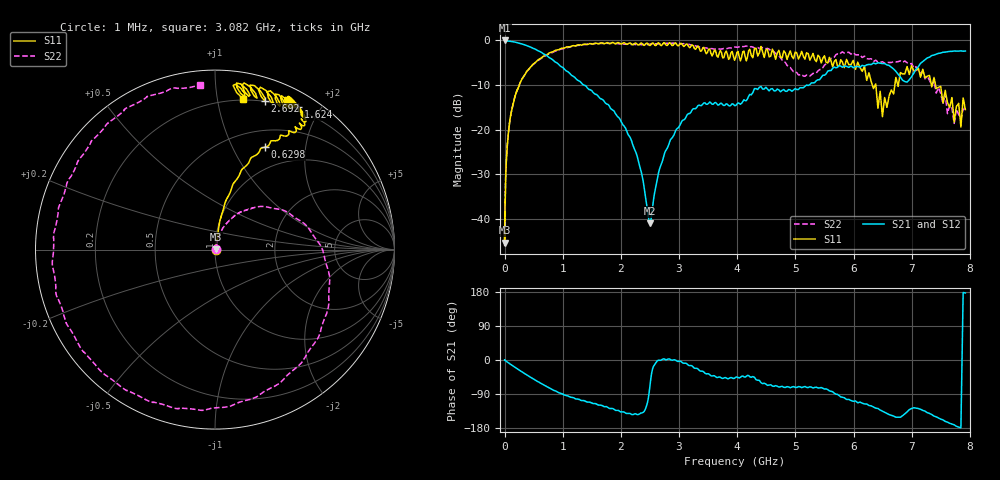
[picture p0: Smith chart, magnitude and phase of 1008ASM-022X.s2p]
!s-Parameter Generated by FASTRON Sdn. Bhd.
!FASTRON P/N : 1008ASM-022X
!Keysight Technologies: E5071C_MY46733604_B.14.02
!Date: Tue Nov 21 11:10:33 2023
!Version  :Rev00  Wed Nov 22 15:46:55 2023
!Data & Calibration Information:
!Freq  S11:SOLT2(ON)  S21:SOLT2(ON)  S12:SOLT2(ON)  S22:SOLT2(ON)
!PortZ  Port1:50+j0  Port2:50+j0
!When reading reference impedance value at option line is always used.
! Remarks : This data is being provided solely for informational purposes.
# Hz S dB R 50
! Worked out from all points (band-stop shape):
!   1599 points, 1 MHz to 7.923 GHz, reference 50 ohm
!   highest |S21| = -0.01 dB at 6.301 MHz (marker M1); lowest = -41.0 dB at 2.502 GHz (marker M2)
!   |S21| within 3 dB of the highest: start of sweep to 669.7 MHz; 7.437 GHz to end of sweep
!   lowest |S11| = -45.3 dB at 1.505 MHz (marker M3), VSWR 1.01, Z = 50.5 + j0.0847 ohm
!   |S11| at or under -10 dB: start of sweep to 252.1 MHz; 6.383 GHz to 6.71 GHz (327.3 MHz wide, 5 % of centre); 7.409 GHz to end of sweep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
!   |S22| runs from -46.1 to -0.6 dB; largest |S21 - S12| = 0.013
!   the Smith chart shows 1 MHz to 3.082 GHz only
!   S11 on the Smith chart (normalised r, x): 1 MHz: 1.01, +0.00; 629.8 MHz: 0.71, +1.34; 1.624 GHz: 0.17, +1.73; 2.692 GHz: 0.20, +1.37; 3.082 GHz: 0.19, +1.18
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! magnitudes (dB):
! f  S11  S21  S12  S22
! 1 MHz  -42.6  -0.1  -0.1  -43.0
! 1.505 MHz  -45.3  -0.1  -0.1  -44.3
! 4.479 MHz  -40.7  -0.1  -0.1  -41.0
! 6.301 MHz  -38.1  0.0  -0.1  -41.6
! 19.95 MHz  -30.6  -0.1  -0.1  -30.2
! 89.01 MHz  -18.2  -0.2  -0.2  -18.2
! 398.5 MHz  -6.7  -1.3  -1.3  -6.7
! 629.8 MHz  -4.0  -2.6  -2.6  -4.0
! 1.624 GHz  -0.8  -12.7  -12.8  -0.7
! 1.784 GHz  -0.6  -14.4  -14.5  -0.7
! 2.146 GHz  -0.6  -21.5  -21.5  -0.9
! 2.502 GHz  -1.1  -41.0  -41.0  -0.8
! 2.575 GHz  -0.9  -34.5  -34.6  -0.8
! 2.692 GHz  -1.2  -27.8  -27.9  -0.7
! 3.082 GHz  -1.4  -17.8  -17.8  -0.7
! 4.437 GHz  -2.6  -10.9  -10.9  -1.6
! 5.164 GHz  -4.2  -10.3  -10.3  -8.1
! 5.841 GHz  -6.1  -5.7  -5.7  -2.8
! 6.496 GHz  -17.1  -5.2  -5.2  -4.8
! 6.805 GHz  -7.2  -8.2  -8.2  -4.6
! 7.19 GHz  -6.5  -4.8  -4.7  -7.0
! 7.923 GHz  -15.5  -2.4  -2.4  -15.4
